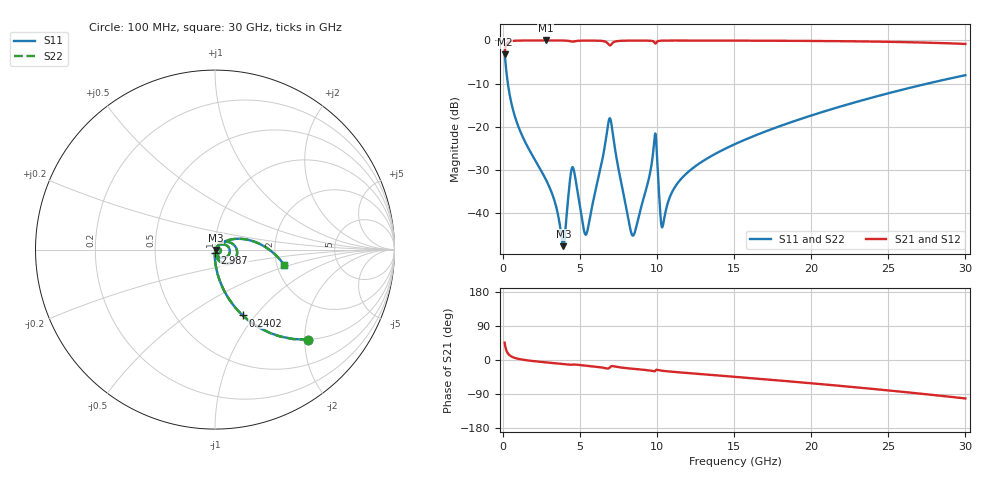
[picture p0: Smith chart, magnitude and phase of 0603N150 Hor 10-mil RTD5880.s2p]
# GHz S MA R 50
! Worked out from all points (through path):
!   3201 points, 100 MHz to 30 GHz, reference 50 ohm
!   highest |S21| = -0.02 dB at 2.763 GHz (marker M1); lowest = -3.2 dB at 100 MHz (marker M2)
!   group delay of S21, straight-line fit = 9.63 ps
!   lowest |S11| = -47.6 dB at 3.912 GHz (marker M3), VSWR 1.01, Z = 50.4 - j0.191 ohm
!   |S11| at or under -10 dB: 312.3 MHz to 27.53 GHz (27.22 GHz wide, 196 % of centre)
!   |S22| runs from -47.6 to -2.8 dB; largest |S21 - S12| = 0
!   S11 on the Smith chart (normalised r, x): 100 MHz: 0.99, -2.08; 240.2 MHz: 0.99, -0.86; 2.987 GHz: 1.00, -0.04; 30 GHz: 2.20, -0.45
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0.1  0.7224 -44.0  0.6912 46.0  0.6912 46.0  0.7224 -44.0
0.2401562  0.3983 -67.1  0.9168 22.8  0.9168 22.8  0.3983 -67.1
0.959625  0.1044 -86.2  0.9937 3.3  0.9937 3.3  0.1044 -86.2
2.762969  0.02487 -92.7  0.9981 -6.2  0.9981 -6.2  0.02487 -92.7
2.987219  0.02049 -92.5  0.9981 -7.1  0.9981 -7.1  0.02049 -92.5
3.91225  0.004162 -27.1  0.996 -10.7  0.996 -10.7  0.004162 -27.1
4.491562  0.03405 -13.8  0.9659 -12.4  0.9659 -12.4  0.03405 -13.8
5.089563  0.009251 -52.8  0.9927 -13.7  0.9927 -13.7  0.009251 -52.8
5.472656  0.006285 15.7  0.9945 -15.3  0.9945 -15.3  0.006285 15.7
6.911594  0.1254 -10.6  0.8761 -20.2  0.8761 -20.2  0.1254 -10.6
8.387906  0.005557 -24.8  0.9943 -23.0  0.9943 -23.0  0.005557 -24.8
9.378344  0.02196 46.6  0.9934 -26.9  0.9934 -26.9  0.02196 46.6
9.8175  0.07066 17.9  0.951 -29.9  0.951 -29.9  0.07066 17.9
9.938969  0.06723 -45.3  0.9362 -26.0  0.9362 -26.0  0.06723 -45.3
10.06978  0.02455 -70.0  0.9819 -26.6  0.9819 -26.6  0.02455 -70.0
10.22862  0.008678 -46.0  0.9916 -27.9  0.9916 -27.9  0.008678 -46.0
10.36878  0.007195 4.2  0.9938 -28.6  0.9938 -28.6  0.007195 4.2
11.6115  0.02565 48.0  0.9956 -33.2  0.9956 -33.2  0.02565 48.0
15.05  0.06313 41.7  0.9936 -44.5  0.9936 -44.5  0.06313 41.7
20.03956  0.1359 26.3  0.9853 -61.5  0.9853 -61.5  0.1359 26.3
25.01978  0.245 8.2  0.9628 -80.3  0.9628 -80.3  0.245 8.2
30  0.3959 -12.6  0.91 -101.5  0.91 -101.5  0.3959 -12.6
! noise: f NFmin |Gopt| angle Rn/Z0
0.1  0.0003084  0.9227  0.471  0.0008831
3.417  0.003927  0.8052  9.459  0.00416
6.743  0.02918  0.9445  18.57  0.1146
10.06  0.0205  0.8865  27.58  0.037
13.39  0.01075  0.737  36.34  0.007396
16.7  0.01268  0.7265  44.91  0.007903
20.03  0.01485  0.7238  53.29  0.008581
23.35  0.01726  0.726  61.41  0.009334
26.67  0.01997  0.732  69.33  0.01016
30  0.02306  0.7412  77.03  0.01109
